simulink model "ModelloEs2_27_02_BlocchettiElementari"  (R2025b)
settings: Solver=FixedStepAuto  StartTime=0.0  StopTime=Tsim  FixedStep=Tc  RelTol=1e-3
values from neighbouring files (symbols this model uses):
  a = 25    [ScriptEs2_27_02.m]    (also in ScriptEs2_26_02.m = 5)
  x0 = 2    [ScriptEs2_27_02.m]    (also in ScriptEs2_26_02.m = 1)
  y0 = -1    [ScriptEs2_27_02.m]    (also in ScriptEs2_26_02.m)
  y0punto = 1    [ScriptEs2_27_02.m]

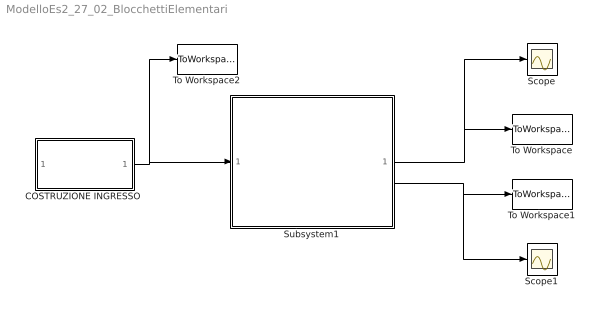
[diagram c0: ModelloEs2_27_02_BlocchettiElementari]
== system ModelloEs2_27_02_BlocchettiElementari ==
  "COSTRUZIONE INGRESSO " : Subsystem
  Scope : Scope
  Scope1 : Scope
  Subsystem1 : Subsystem
  To Workspace : ToWorkspace  VariableName=x  SaveFormat=Timeseries  SampleTime=-1
  To Workspace1 : ToWorkspace  VariableName=y  SaveFormat=Timeseries  SampleTime=-1
  To Workspace2 : ToWorkspace  VariableName=u  SaveFormat=Timeseries  SampleTime=-1
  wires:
  "COSTRUZIONE INGRESSO "/1("u(t) ") -> Subsystem1/1("u(t) "), To Workspace2/1
  Subsystem1/2("y(t) ") -> Scope1/1, To Workspace1/1
  Subsystem1/1("x(t) ") -> Scope/1, To Workspace/1

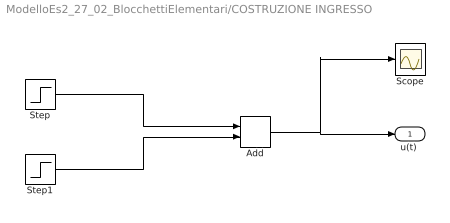
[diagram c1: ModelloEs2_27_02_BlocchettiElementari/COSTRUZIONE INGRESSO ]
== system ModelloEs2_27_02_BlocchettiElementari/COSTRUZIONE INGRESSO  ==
  Add : Sum
  Scope : Scope
  Step : Step  Time=3  Before=2  After=4  SampleTime=0
  Step1 : Step  Time=6  After=0.5  SampleTime=0
  "u(t) " : Outport  VectorParamsAs1DForOutWhenUnconnected=off
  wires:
  Add/1 -> Scope/1, "u(t) "/1
  Step/1 -> Add/1
  Step1/1 -> Add/2

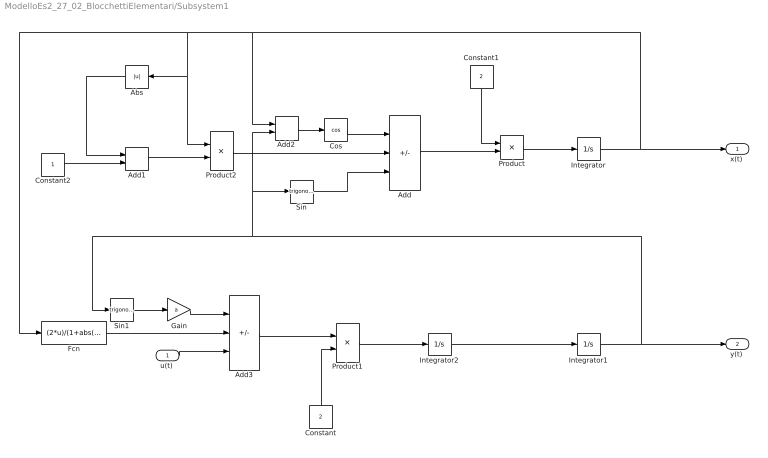
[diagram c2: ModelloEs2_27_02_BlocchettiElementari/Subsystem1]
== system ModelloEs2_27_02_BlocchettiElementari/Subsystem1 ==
  "u(t) " : Inport
  Abs : Abs
  Add : Sum  Inputs=+-+
  Add1 : Sum
  Add2 : Sum
  Add3 : Sum  Inputs=-++
  Constant : Constant  Value=2
  Constant1 : Constant  Value=2
  Constant2 : Constant
  Cos : Trigonometry  Operator=cos
  Fcn : Fcn  Expr=(2*u)/(1+abs(u))
  Gain : Gain  Gain=a
  Integrator : Integrator  InitialCondition=x0
  Integrator1 : Integrator  InitialCondition=y0
  Integrator2 : Integrator  InitialCondition=y0punto
  Product : Product
  Product1 : Product  Inputs=*/
  Product2 : Product  Inputs=*/
  Sin : Trigonometry
  Sin1 : Trigonometry
  "x(t) " : Outport  VectorParamsAs1DForOutWhenUnconnected=off
  "y(t) " : Outport  Port=2  VectorParamsAs1DForOutWhenUnconnected=off
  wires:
  Integrator/1 -> Add2/1, Product2/1, Abs/1, Fcn/1, "x(t) "/1
  Integrator1/1 -> Sin1/1, Add2/2, Sin/1, "y(t) "/1
  Integrator2/1 -> Integrator1/1
  Product/1 -> Integrator/1
  Product1/1 -> Integrator2/1
  Constant/1 -> Product1/2
  Constant1/1 -> Product/1
  Add/1 -> Product/2
  Sin/1 -> Add/3
  Product2/1 -> Add/2
  Add1/1 -> Product2/2
  Abs/1 -> Add1/1
  Constant2/1 -> Add1/2
  Cos/1 -> Add/1
  Add2/1 -> Cos/1
  Add3/1 -> Product1/1
  "u(t) "/1 -> Add3/3
  Sin1/1 -> Gain/1
  Gain/1 -> Add3/1
  Fcn/1 -> Add3/2
